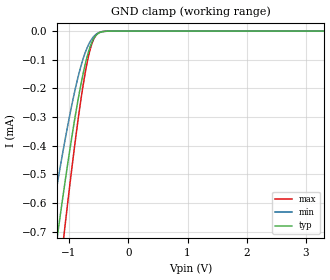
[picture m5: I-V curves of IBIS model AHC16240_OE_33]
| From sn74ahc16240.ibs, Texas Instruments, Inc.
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[Model]   AHC16240_OE_33
Model_type  Input
Vinl = 0.9
Vinh = 2.34
| variable   typ   min   max
C_comp   0.84pF   0.76pF   0.93pF
[Temperature Range]   40   100   -40
| Ambient temperature   25   85   -40
[Voltage range]   3.3   3   3.6
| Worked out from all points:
|   GND clamp passes 1 mA (typ) near -1.38 V on its own axis
[GND Clamp]
| AHC16240_OE_33
|   Voltage   I(typ)   I(min)   I(max)
-5.5V     -8.851mA   -7.354mA   -10.02mA
-1.375V   -991uA     -755.7uA   -1.257mA
-1.32V    -904.2uA   -685uA     -1.15mA
-1.175V   -682.2uA   -505uA     -875.6uA
-1.085V   -550.6uA   -399.5uA   -710.3uA
-1.065V   -522.1uA   -376.9uA   -674.3uA
-895mV    -295.8uA   -201.7uA   -383.4uA
-800mV    -186.7uA   -122.7uA   -239.7uA
-730mV    -118.5uA   -76.84uA   -149uA
-620mV    -41.44uA   -28.88uA   -47.61uA
-505mV    -7.613uA   -6.114uA   -6.771uA
3.3V      1.837nA    303.9pA    8.84nA
